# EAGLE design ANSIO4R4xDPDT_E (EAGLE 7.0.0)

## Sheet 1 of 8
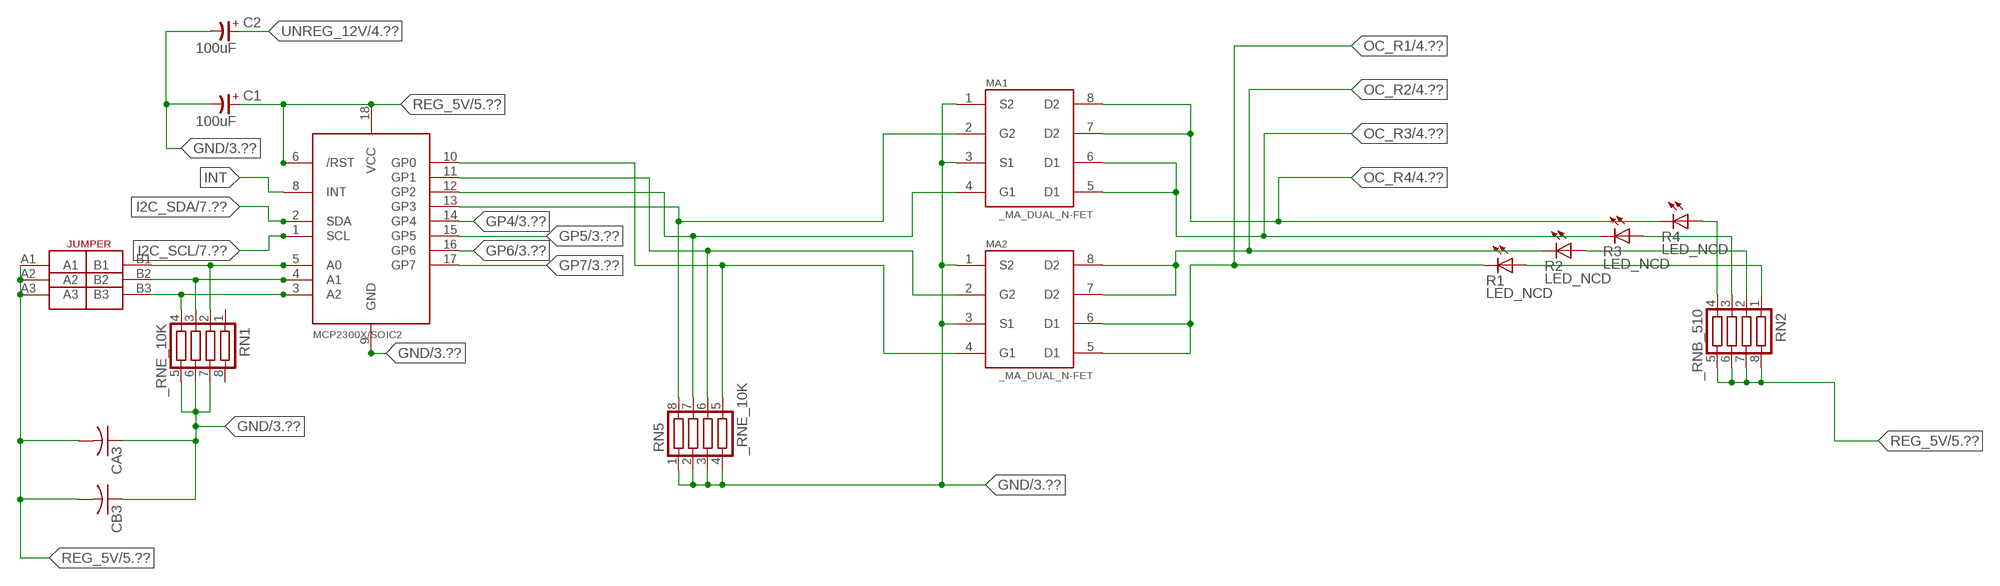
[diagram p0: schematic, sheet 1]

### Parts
C1  100uF  CP-E-025X060  [E-025X060]
C2  100uF  CP-E-025X060  [E-025X060]
CA3  CC1206KRX7R9BB104C1206K  [CC1206KRX7R9BB104]
CB3  TMK316F106ZL-TC1206K  [TMK316F106ZL-T]
IC2  MCP2300X/SO  [SO18W]
MA1  _MA_DUAL_N-FET  [_MA_DUAL_N-FET]
MA2  _MA_DUAL_N-FET  [_MA_DUAL_N-FET]
R1  LED_NCD  [CHIPLED_0603]
R2  LED_NCD  [CHIPLED_0603]
R3  LED_NCD  [CHIPLED_0603]
R4  LED_NCD  [CHIPLED_0603]
RN1  _RNE_10K  [RNE]
RN2  _RNB_510  [RNB]
RN5  _RNE_10K  [RNE]
U$18  JUMPER_3X2  [JUMPER_3X2]

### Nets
GND: C1.- C2.- CA3.1 CB3.1 IC2.9(GND) MA1.1(S2) MA1.3(S1) MA2.1(S2) MA2.3(S1) RN1.5 RN1.6 RN1.7 RN5.1 RN5.2 RN5.3 RN5.4 ; also sheet 3,5,6,7,8
GP4: IC2.14(GP4) ; also sheet 3
GP5: IC2.15(GP5) ; also sheet 3
GP6: IC2.16(GP6) ; also sheet 3
GP7: IC2.17(GP7) ; also sheet 3
I2C_SCL: IC2.1(SCL) ; also sheet 7,8
I2C_SDA: IC2.2(SDA) ; also sheet 7,8
INT: IC2.8(INT)
N$6: IC2.5(A0) RN1.2 U$18.B1
N$7: IC2.4(A1) RN1.3 U$18.B2
N$8: IC2.3(A2) RN1.4 U$18.B3
N$20: IC2.13(GP3) MA1.2(G2) RN5.8
N$21: IC2.12(GP2) MA1.4(G1) RN5.7
N$22: IC2.11(GP1) MA2.2(G2) RN5.6
N$23: IC2.10(GP0) MA2.4(G1) RN5.5
N$29: R4.A RN2.4
N$30: R3.A RN2.3
N$31: R2.A RN2.2
N$32: R1.A RN2.1
OC_R1: MA2.5(D1) MA2.6(D1) R1.C ; also sheet 4
OC_R2: MA2.7(D2) MA2.8(D2) R2.C ; also sheet 4
OC_R3: MA1.5(D1) MA1.6(D1) R3.C ; also sheet 4
OC_R4: MA1.7(D2) MA1.8(D2) R4.C ; also sheet 4
REG_5V: C1.+ CA3.2 CB3.2 IC2.6(/RST) IC2.18(VCC) RN2.5 RN2.6 RN2.7 RN2.8 U$18.A1 U$18.A2 U$18.A3 ; also sheet 5,6,7,8
UNREG_12V: C2.+ ; also sheet 4,5
Unconnected: RN1.1 RN1.8

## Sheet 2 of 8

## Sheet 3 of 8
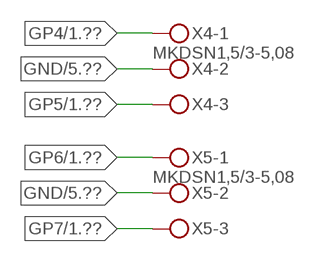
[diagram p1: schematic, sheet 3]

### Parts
X4  MKDSN1,5/3-5,08  [MKDSN1,5/3-5,08]
X5  MKDSN1,5/3-5,08  [MKDSN1,5/3-5,08]

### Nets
GND: X4.2 X5.2 ; also sheet 1,5,6,7,8
GP4: X4.1 ; also sheet 1
GP5: X4.3 ; also sheet 1
GP6: X5.1 ; also sheet 1
GP7: X5.3 ; also sheet 1

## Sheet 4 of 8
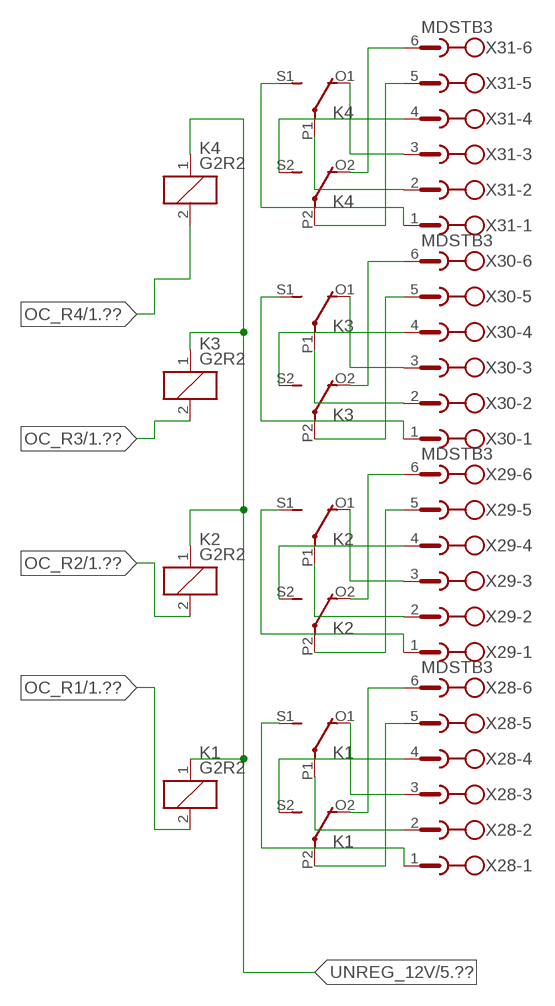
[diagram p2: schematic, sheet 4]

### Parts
K1  G2R2  [G2R2]
K2  G2R2  [G2R2]
K3  G2R2  [G2R2]
K4  G2R2  [G2R2]
X28  MDSTB3  [MDSTB3]
X29  MDSTB3  [MDSTB3]
X30  MDSTB3  [MDSTB3]
X31  MDSTB3  [MDSTB3]

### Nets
N$9: K3.P2(3:COM) X30.5
N$10: K3.O2(3:NC) X30.6
N$11: K4.P2(3:COM) X31.5
N$12: K4.O2(3:NC) X31.6
N$13: K3.S2(3:NO) X30.4
N$14: K4.S2(3:NO) X31.4
N$15: K3.O1(2:NC) X30.3
N$16: K4.O1(2:NC) X31.3
N$17: K4.P1(2:COM) X31.2
N$18: K3.P1(2:COM) X30.2
N$19: K3.S1(2:NO) X30.1
N$24: K4.S1(2:NO) X31.1
N$203: K1.P2(3:COM) X28.5
N$204: K1.O2(3:NC) X28.6
N$205: K1.S2(3:NO) X28.4
N$206: K1.P1(2:COM) X28.2
N$207: K1.O1(2:NC) X28.3
N$208: K1.S1(2:NO) X28.1
N$209: K2.P2(3:COM) X29.5
N$210: K2.O2(3:NC) X29.6
N$211: K2.S2(3:NO) X29.4
N$212: K2.S1(2:NO) X29.1
N$213: K2.P1(2:COM) X29.2
N$214: K2.O1(2:NC) X29.3
OC_R1: K1.2(1:C2) ; also sheet 1
OC_R2: K2.2(1:C2) ; also sheet 1
OC_R3: K3.2(1:C2) ; also sheet 1
OC_R4: K4.2(1:C2) ; also sheet 1
UNREG_12V: K1.1(1:C1) K2.1(1:C1) K3.1(1:C1) K4.1(1:C1) ; also sheet 1,5

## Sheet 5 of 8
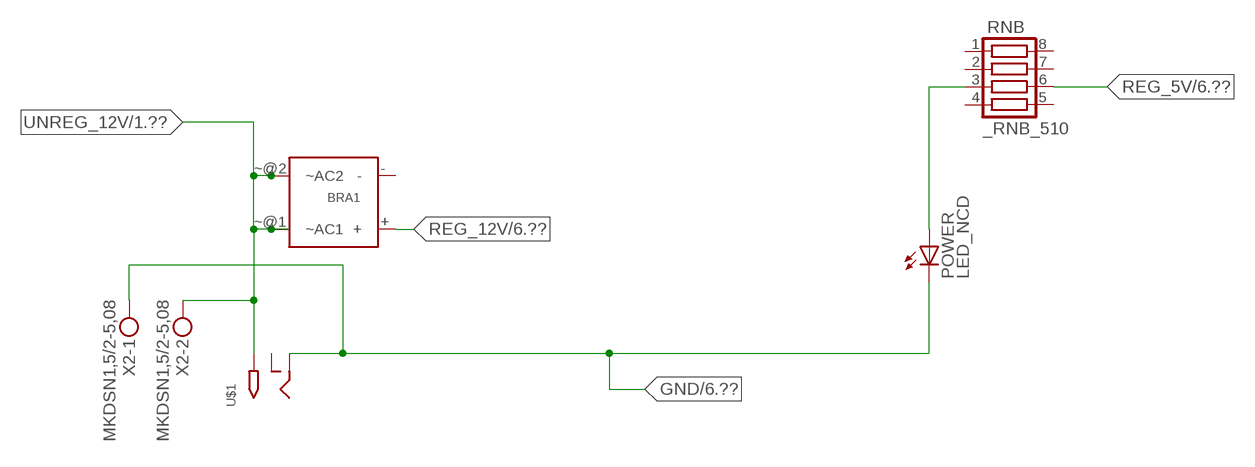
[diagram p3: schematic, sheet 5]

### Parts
BRA1  MB2S_  [MB2S]
POWER  LED_NCD  [CHIPLED_0603]
RNB  _RNB_510  [RNB]
U$1  2.1MMJACK  [PJ-102A]
X2  MKDSN1,5/2-5,08  [MKDSN1,5/2-5,08]

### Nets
GND: POWER.C U$1.RING X2.1 ; also sheet 1,3,6,7,8
N$2: POWER.A RNB.3
REG_5V: RNB.6 ; also sheet 1,6,7,8
REG_12V: BRA1.+ ; also sheet 6
UNREG_12V: BRA1.~@1(~AC1) BRA1.~@2(~AC2) U$1.TIP X2.2 ; also sheet 1,4
Unconnected: BRA1.- RNB.1 RNB.2 RNB.4 RNB.5 RNB.7 RNB.8 U$1.RING_SW

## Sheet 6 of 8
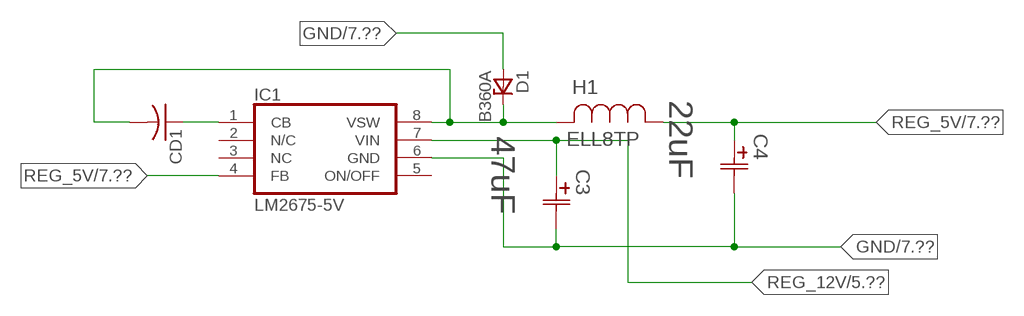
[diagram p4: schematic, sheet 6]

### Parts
C3  47uF  490-5463-6-NDCAP  [C2917(7343)-Y]
C4  22uF  490-5463-6-NDCAP  [C2917(7343)-Y]
CD1  _CD_10NF_50VC1206K  [_CD_10NF_50V]
D1  B360A  [DO214AC_ZENER]
H1  ELL8TP  [IND_ELL8TP]
IC1  LM2675-5V  LM2675  [SO-8]

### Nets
GND: C3.2(C2) C4.2(C2) D1.A IC1.6(GND) ; also sheet 1,3,5,7,8
N$1: CD1.2 D1.C H1.2 IC1.8(VSW)
N$3: CD1.1 IC1.1(CB)
REG_5V: C4.1(C1) H1.1 IC1.4(FB) ; also sheet 1,5,7,8
REG_12V: C3.1(C1) IC1.7(VIN) ; also sheet 5
Unconnected: IC1.2(N/C) IC1.5(ON/OFF)

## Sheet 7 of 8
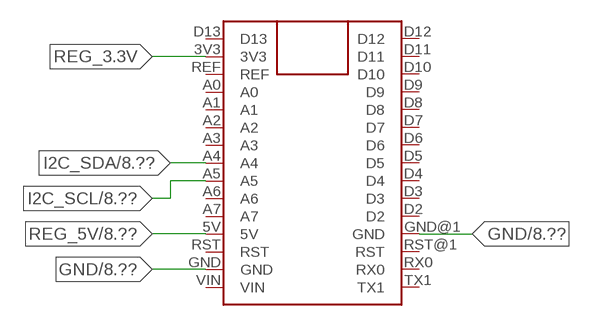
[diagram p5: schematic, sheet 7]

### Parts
FOR_NANO  ARDUINO_NANO  [ARDUINO_NANO]

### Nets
GND: FOR_NANO.GND FOR_NANO.GND@1(GND) ; also sheet 1,3,5,6,8
I2C_SCL: FOR_NANO.A5 ; also sheet 1,8
I2C_SDA: FOR_NANO.A4 ; also sheet 1,8
REG_3.3V: FOR_NANO.3V3
REG_5V: FOR_NANO.5V ; also sheet 1,5,6,8
Unconnected: FOR_NANO.A0 FOR_NANO.A1 FOR_NANO.A2 FOR_NANO.A3 FOR_NANO.A6 FOR_NANO.A7 FOR_NANO.D2 FOR_NANO.D3 FOR_NANO.D4 FOR_NANO.D5 FOR_NANO.D6 FOR_NANO.D7 FOR_NANO.D8 FOR_NANO.D9 FOR_NANO.D10 FOR_NANO.D11 FOR_NANO.D12 FOR_NANO.D13 FOR_NANO.REF FOR_NANO.RST FOR_NANO.RST@1(RST) FOR_NANO.RX0 FOR_NANO.TX1 FOR_NANO.VIN

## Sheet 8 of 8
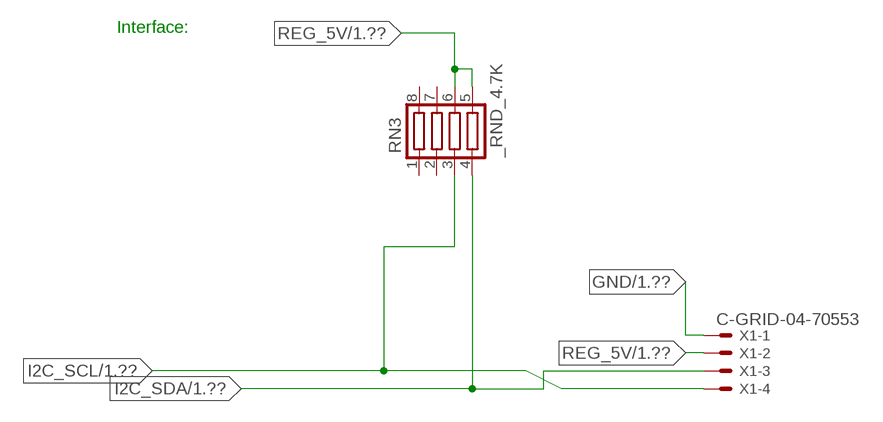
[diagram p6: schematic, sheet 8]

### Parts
RN3  _RND_4.7K  [RND]
X1  C-GRID-04-70553  [70553-04]

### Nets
GND: X1.1 ; also sheet 1,3,5,6,7
I2C_SCL: RN3.3 X1.4 ; also sheet 1,7
I2C_SDA: RN3.4 X1.3 ; also sheet 1,7
REG_5V: RN3.5 RN3.6 X1.2 ; also sheet 1,5,6,7
Unconnected: RN3.1 RN3.2 RN3.7 RN3.8

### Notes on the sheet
- Interface:

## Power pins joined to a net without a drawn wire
NC: IC1.3(NC)

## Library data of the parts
BRA1 = NCD_ULTIMATE_LIBRARY:MB2S: Bridge Rectifier BRA MB2S 200V 500ma Digikey MB2S-TPMSTR-ND/MB2S-TP
C1 C2 = NCD_ULTIMATE_LIBRARY:CP-: Capacitors All Kinds POLARIZED CAP
C3 C4 = NCD_ULTIMATE_bhaskar:490-5463-6-ND: NCD CAP
CA3 = NCD_ULTIMATE_LIBRARY:CC1206KRX7R9BB104: Capacitor CA .1uF 50V SMT C1206K CC1206KRX7R9BB104
CB3 = NCD_ULTIMATE_LIBRARY:TMK316F106ZL-T: Capacitor CB 10uF SMT 1206 TMK316F106ZL-T
CD1 = NCD_ULTIMATE_LIBRARY:_CD_10NF_50V: Capacitor 10nF SMT
D1 = NCD_ULTIMATE_bhaskar:B360A: NCD DIODE B350A/B360A
FOR_NANO = NCD_ULTIMATE_CONNECTORS:ARDUINO_NANO
H1 = NCD_ULTIMATE_bhaskar:ELL8TP: NCD coil
IC1 = NCD_ULTIMATE_bhaskar:LM2675: LM2675 NCD http://www.ti.com/lit/ds/symlink/lm2675.pdf
IC2 = NCD_ULTIMATE_LIBRARY:MCP2300X: Semiconductor Port Expander I/O 8-Bit I2C MCP23008 Inexpensive i2c i/o expander - 8 general purpose i/o pins with optional pullups
K1-K4 = NCD_ULTIMATE_LIBRARY:G2R2: RELAY 2 x switch, Omron
MA1 MA2 = NCD_ULTIMATE_LIBRARY:_MA_DUAL_N-FET: FET Dual N-Channel 8-SOIC NMOSFET Digikey 785-1064-2-ND/AO4842
POWER = NCD_ULTIMATE_bhaskar:LED_NCD
R1-R4 = NCD_ULTIMATE_LIBRARY:LED_NCD: LED Digikey 754-1132-2-ND/APT2012SRCPRV
RN1 RN5 = NCD_ULTIMATE_LIBRARY:_RNE_10K: Resistor Array RNE SMT 10K x 4 Single Resistor Source: http://www.ctscorp.com/components/Datasheets/CTSChipArrayDs.pdf Digikey 742C083103JPTR-ND/742C083103JP; OC_FARNELL: unknown; OC_NEWARK: unknown
RN2 RNB = NCD_ULTIMATE_LIBRARY:_RNB_510: Resistor Array RNB SMT 510 x 4 Single Resistor Source: http://www.ctscorp.com/components/Datasheets/CTSChipArrayDs.pdf Digikey 742C083511JPTR-ND/ 742C083511JP; OC_FARNELL: unknown; OC_NEWARK: unknown
RN3 = NCD_ULTIMATE_LIBRARY:_RND_4.7K: Resistor Array RND SMT 4.7K x 4 Single Resistor Source: http://www.ctscorp.com/components/Datasheets/CTSChipArrayDs.pdf Digikey 742C083472JPTR-ND/742C083472JP; OC_FARNELL: unknown; OC_NEWARK: unknown
U$1 = NCD_ULTIMATE_CONNECTORS:2.1MMJACK: 2.1mm x 5.5mm DC jack with internal switch. Digikey part #PJ-102A, 4UCON part #05537 By microbuilder.eu
U$18 = NCD_ULTIMATE_CONNECTORS:JUMPER_3X2
X1 = NCD_ULTIMATE_CONNECTORS:C-GRID-04: CONNECTOR 4-Pos I2C wire to board 2.54 mm (0.100") pitch header Digikey WM1342-ND/0015912045; OC_FARNELL: unknown; OC_NEWARK: unknown
X2 = NCD_ULTIMATE_CONNECTORS:MKDSN1,5/2-5,08: MKDSN 1,5/ 2-5,08 Printklemme
X4 X5 = NCD_ULTIMATE_CONNECTORS:MKDSN1,5/3-5,08: MKDSN 1,5/ 3-5,08 Printklemme Nennstrom: 13,5 A Nennspannung: 250 V Rastermaß: 5,08 mm Polzahl: 3 Anschlussart: Schraubanschluss Montage: Löten Anschlussrichtung Leiter/Platine: 0 ° Artikelnummer: 1729131 Source: http://eshop.phoenixcontact.com .. 1729131.pdf
X28-X31 = NCD_ULTIMATE_LIBRARY:MDSTB3: PHOENIX

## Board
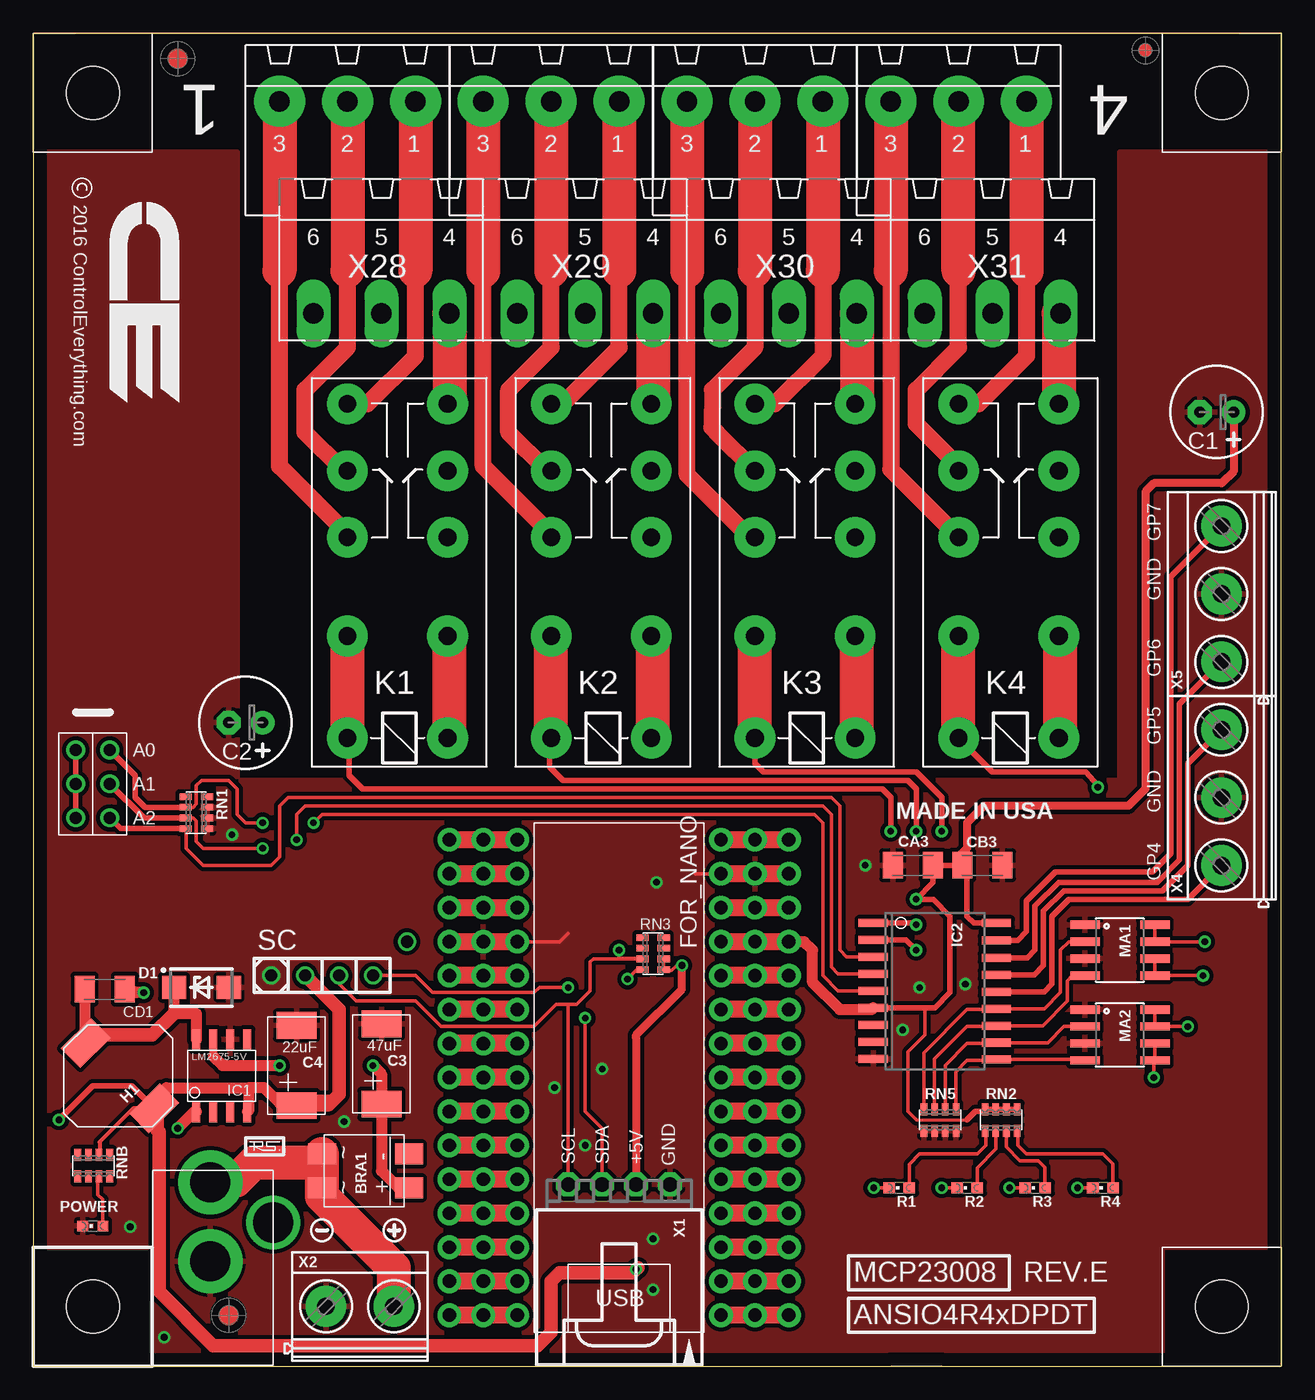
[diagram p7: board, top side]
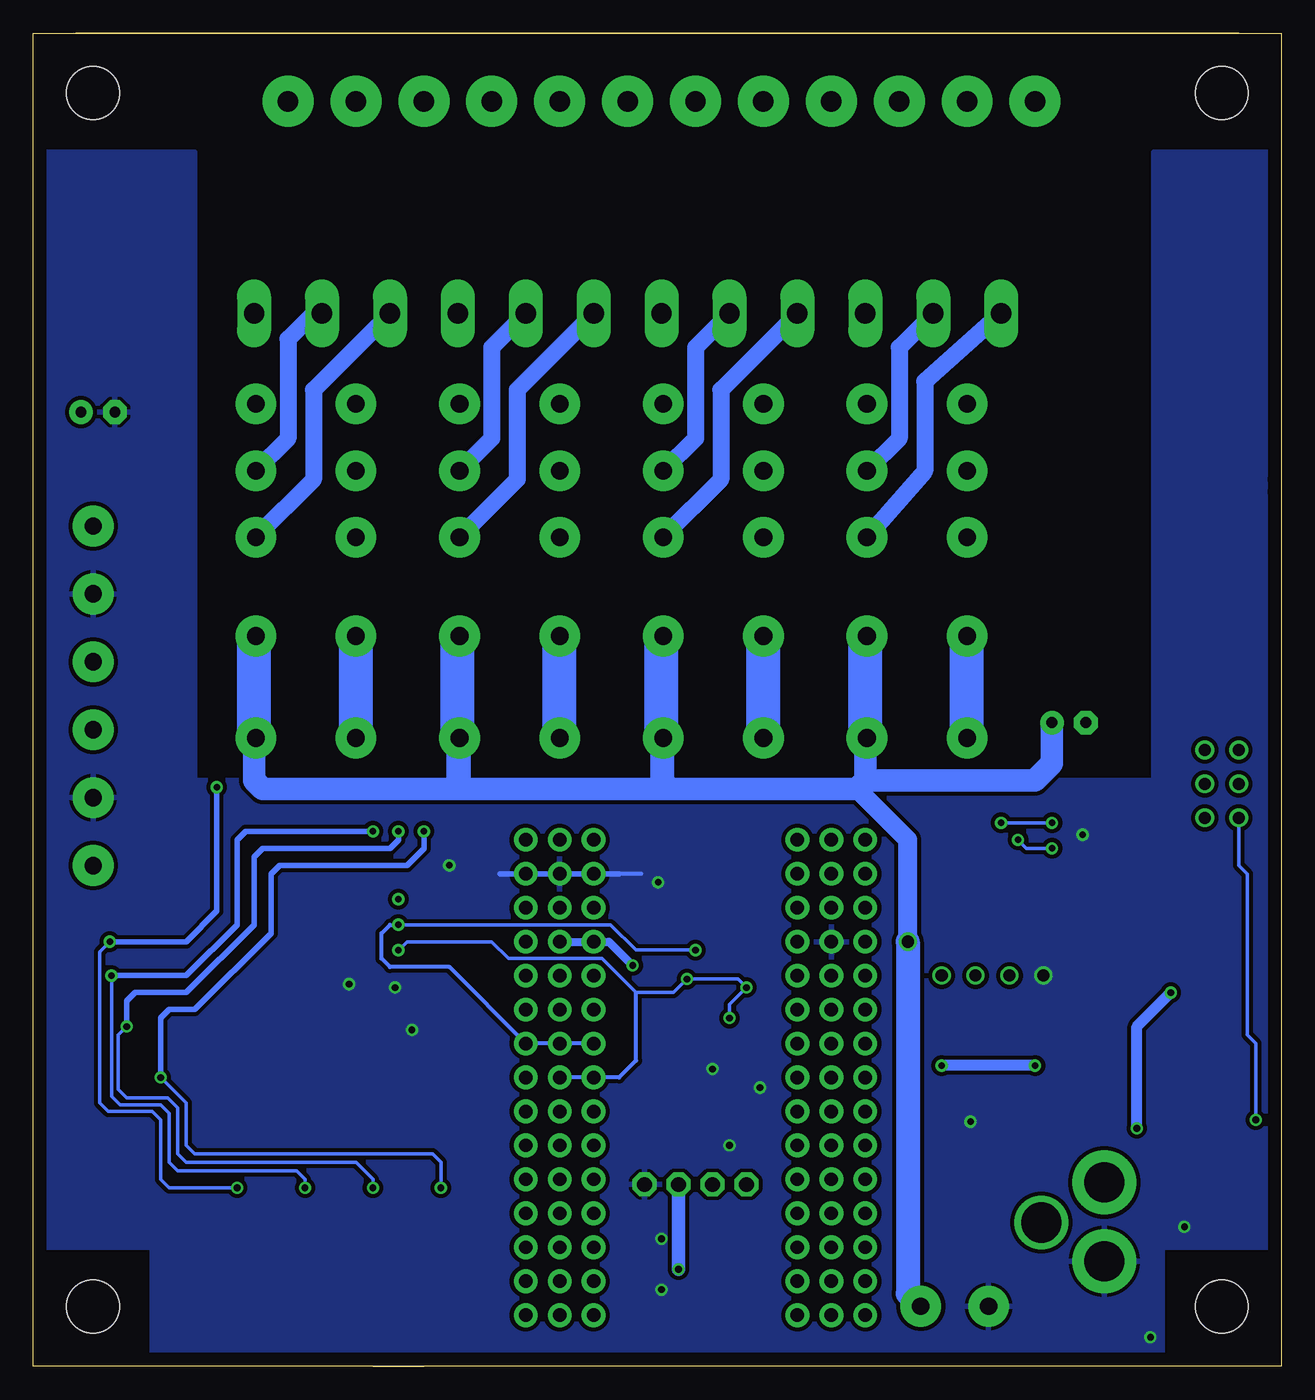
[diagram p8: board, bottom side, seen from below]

Size 93.34 x 99.7 mm. Coordinates in mm from the lower left corner, seen from the top.
Outline: 0,66.34 0,65.41
Outline: 0,65.41 0,0 64.14,0
Outline: 64.14,0 93.34,0 93.34,99.7 0,99.7 0,65.41
Outline: 3.17,99.7 90.17,99.7
Outline: 67.94,0 64.14,0
Copper layers (1*16): Top 0.035mm / dielectric 1.5mm / Bottom 0.035mm
Design rules "default": minimum track width 10mil, minimum drill 24mil, track to track 8mil, track to pad 8mil, pad to pad 8mil, via to via 8mil, smd to smd 8mil, copper to edge 40mil, drill to drill 8mil, minimum pad ring 10mil, minimum via ring 8mil, stop-mask expansion 4mil, vias tented up to drill 0mil, thermal gap 10mil
Holes 3.96 mm at 4.45,4.45 4.45,4.45 4.45,4.45

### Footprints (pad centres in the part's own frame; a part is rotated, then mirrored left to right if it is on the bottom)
MB2S = smd 1.55 x 2.1: + 0,-6.5; - 2.54,-6.5; ~@1 0,0; ~@2 2.54,0
E-025X060 = drill 0.813 pad 1.778: + -1.27,0 | drill 0.813 pad 1.778 octagon: - 1.27,0
C2917(7343)-Y = smd 2 x 3: 1 -3,0; 2 3,0
CC1206KRX7R9BB104 = smd 1.5 x 2: 1 -1.5,0; 2 1.5,0
TMK316F106ZL-T = smd 1.5 x 2: 1 -1.5,0; 2 1.5,0
_CD_10NF_50V = smd 1.5 x 2: 1 -1.5,0; 2 1.5,0
DO214AC_ZENER = smd 1.8 x 1.7: A 2.05,0; C -2.05,0
ARDUINO_NANO = drill 1 pad 1.778: 3V1 -2.54,-2.54; 3V3 0,-2.54; 5V 0,-27.94; 5V1 -2.54,-27.94; A0 0,-7.62; A1 0,-10.16; A2 0,-12.7; A3 0,-15.24; A4 0,-17.78; A5 0,-20.32; A6 0,-22.86; A7 0,-25.4; A8 -2.54,-7.62; A9 -2.54,-10.16; A10 -2.54,-12.7; A11 -2.54,-15.24; A12 -2.54,-17.78; A13 -2.54,-20.32; A14 -2.54,-22.86; A15 -2.54,-25.4; D1 -2.54,0; D2 20.32,-25.4; D3 20.32,-22.86; D4 20.32,-20.32; D5 20.32,-17.78; D6 20.32,-15.24; D7 20.32,-12.7; D8 20.32,-10.16; D9 20.32,-7.62; D10 20.32,-5.08; D11 20.32,-2.54; D12 20.32,0; D13 0,0; D14 22.86,0; D15 22.86,-2.54; D16 22.86,-5.08; D17 22.86,-7.62; D18 22.86,-10.16; D19 22.86,-12.7; D20 22.86,-15.24; D21 22.86,-17.78; D22 22.86,-20.32; D23 22.86,-22.86; D24 22.86,-25.4; GND 0,-33.02; GND1 -2.54,-33.02; GND@1 20.32,-27.94; GND@2 22.86,-27.94; P$16 2.54,0; P$17 2.54,-2.54; P$18 2.54,-5.08; P$19 2.54,-7.62; P$20 2.54,-10.16; P$21 2.54,-12.7; P$22 2.54,-15.24; P$23 2.54,-17.78; P$24 2.54,-20.32; P$25 2.54,-22.86; P$26 2.54,-25.4; P$27 2.54,-27.94; P$28 2.54,-30.48; P$29 2.54,-33.02; P$30 2.54,-35.56; P$31 17.78,0; P$32 17.78,-2.54; P$33 17.78,-5.08; P$34 17.78,-7.62; P$35 17.78,-10.16; P$36 17.78,-12.7; P$37 17.78,-15.24; P$38 17.78,-17.78; P$39 17.78,-20.32; P$40 17.78,-22.86; P$41 17.78,-25.4; P$42 17.78,-27.94; P$43 17.78,-30.48; P$44 17.78,-33.02; P$45 17.78,-35.56; REF 0,-5.08; REF1 -2.54,-5.08; RST 0,-30.48; RST1 -2.54,-30.48; RST@1 20.32,-30.48; RST@2 22.86,-30.48; RX0 20.32,-33.02; RX1 22.86,-33.02; TX1 20.32,-35.56; TX2 22.86,-35.56; VIN 0,-35.56; VIN1 -2.54,-35.56
IND_ELL8TP = smd 2.054 x 3.2 rotated 45: 1 -2.442,-2.696; 2 2.442,2.442
SO-8 = smd 0.6 x 1.55: 1 -1.905,-2.69; 2 -0.635,-2.69; 3 0.635,-2.69; 4 1.905,-2.69; 5 1.905,2.71; 6 0.635,2.71; 7 -0.635,2.71; 8 -1.905,2.71
SO18W = smd 0.6 x 2.2: 1 -4.445,-4.6; 2 -3.175,-4.6; 3 -1.905,-4.6; 4 -0.635,-4.6; 5 0.635,-4.6; 6 1.905,-4.6; 7 3.175,-4.6; 8 4.445,-4.6; 9 5.715,-4.6; 10 5.775,4.6; 11 4.505,4.6; 12 3.235,4.6; 13 1.965,4.6; 14 0.695,4.6; 15 -0.575,4.6; 16 -1.845,4.6; 17 -3.145,4.6; 18 -4.445,4.6
G2R2 = drill 1.321 pad 3.048: 1 -2.54,-3.683; 2 -2.54,3.81; 3 5.08,-3.683; 4 5.08,3.81; O1 12.471,3.81; O2 12.471,-3.683; P1 17.45,3.81; P2 17.45,-3.683; S1 22.454,3.81; S2 22.454,-3.683
_MA_DUAL_N-FET = smd 0.61 x 2.21: 1 -1.905,-2.616; 2 -0.635,-2.616; 3 0.635,-2.616; 4 1.905,-2.616; 5 1.905,2.616; 6 0.635,2.616; 7 -0.635,2.616; 8 -1.905,2.616
CHIPLED_0603 = smd 0.8 x 0.8: A 0,-0.75; C 0,0.75
CHIPLED_0603' = smd 0.8 x 0.876: A 0,-0.75; C 0,0.75
RNE = smd 0.5 x 0.9: 1 -1.2,-0.8; 2 -0.4,-0.8; 3 0.4,-0.8; 4 1.2,-0.8; 5 1.2,0.8; 6 0.4,0.8; 7 -0.4,0.8; 8 -1.2,0.8
RNB = smd 0.5 x 0.9: 1 -1.2,-0.8; 2 -0.4,-0.8; 3 0.4,-0.8; 4 1.2,-0.8; 5 1.2,0.8; 6 0.4,0.8; 7 -0.4,0.8; 8 -1.2,0.8
RND = smd 0.5 x 0.9: 1 -1.2,-0.8; 2 -0.4,-0.8; 3 0.4,-0.8; 4 1.2,-0.8; 5 1.2,0.8; 6 0.4,0.8; 7 -0.4,0.8; 8 -1.2,0.8
PJ-102A = drill 3 pad 4.8: RING 0.1,-3.39; TIP 0.1,-9.29 | drill 3 pad 3.251: RING_SW -4.6,-6.29
PCB_MOUNTING_HOLE = hole 3.962: 4.445,4.445
JUMPER_3X2 = drill 0.9: A1 0,5.08; A2 0,2.54; A3 0,0; B1 2.54,5.08; B2 2.54,2.54; B3 2.54,0
70553-04 = drill 1.1 pad 1.778 octagon: 1 -3.81,-7.62; 2 -1.27,-7.62; 3 1.27,-7.62; 4 3.81,-7.62
MKDSN1,5/2-5,08 = drill 1.3 pad 3.048: 1 -2.561,0.025; 2 2.519,0.025
MKDSN1,5/3-5,08 = drill 1.3 pad 3.048: 1 -7.641,0.025; 2 -2.561,0.025; 3 2.519,0.025
MDSTB3 = drill 1.524 pad 3.81: 1 -3.81,-10.795; 2 1.27,-10.795; 3 6.35,-10.795 | drill 1.524 pad 2.54 long: 4 -6.35,5.08; 5 -1.27,5.08; 6 3.81,5.08

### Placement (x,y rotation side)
BRA1  21.59,13.34 90 top
C1  88.52,71.37 180 top
C2  15.88,48.13 180 top
C3  26.04,22.61 90 top
C4  19.68,22.48 90 top
CA3  65.79,37.47 0 top
CB3  70.99,37.47 180 top
CD1  5.33,28.19 180 top
D1  12.57,28.32 0 top
FOR_NANO  53.98,3.81 180 top
H1  6.35,21.72 90 top
IC1  14.1,21.72 0 top
IC2  67.44,28.7 270 top
K1  27.3,49.53 90 top
K2  42.55,49.53 90 top
K3  57.78,49.53 90 top
K4  73.03,49.53 90 top
MA1  81.28,31.12 270 top
MA2  81.28,24.77 270 top
POWER  4.45,10.48 90 top
R1  LED_NCD  [CHIPLED_0603']  64.77,13.34 90 top
R2  LED_NCD  [CHIPLED_0603']  69.85,13.34 90 top
R3  LED_NCD  [CHIPLED_0603']  74.93,13.34 90 top
R4  LED_NCD  [CHIPLED_0603']  80.01,13.34 90 top
RN1  12.19,41.4 270 top
RN2  72.39,18.41 0 top
RN3  46.35,30.86 270 top
RN5  67.82,18.41 0 top
RNB  4.51,14.99 0 top
U$1  13.34,4.45 180 top
U$2  [VISION_REF15]  14.61,3.81 0 top
U$3  [ICON_MINUS]  21.59,10.16 180 top
U$4  PCB_MOUNTING_HOLE  [PCB_MOUNTING_HOLE]  93.34,90.81 90 top
U$5  [ICON_PLUS]  26.99,10.16 90 top
U$6  PCB_MOUNTING_HOLE  [PCB_MOUNTING_HOLE]  93.34,0 90 top
U$11  PCB_MOUNTING_HOLE  [PCB_MOUNTING_HOLE]  8.89,90.81 90 top
U$15  [VISION_REF15]  10.79,97.79 270 top
U$18  3.17,41.02 0 top
U$19  [VISION_REF10]  83.19,98.43 0 top
U$21  [ICON_USA]  64.52,40.89 0 top
X1  43.81,5.97 180 top
X2  24.45,4.45 0 top
X4  88.9,45.09 90 top
X5  88.9,60.32 90 top
X28  24.77,83.82 180 top
X29  40.01,83.82 180 top
X30  55.24,83.82 180 top
X31  70.48,83.82 180 top

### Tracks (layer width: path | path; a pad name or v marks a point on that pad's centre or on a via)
GND  (via drill 0.5, 0.9)
  Top 0.254: 36.2,31.75 39.37,31.75 40.01,32.38 | FOR_NANO.GND@1 32.38,31.75 | 49.53,36.83 56.52,36.83 56.77,36.83
  Top 1.016: X1.1 47.62,13.49
  Bottom 0.254: 51.44,36.83 FOR_NANO.GND
  Bottom 0.305: 47.88,36.83 49.53,36.83 51.44,36.83
  Bottom 0.406: 49.53,36.83 58.42,36.83
  other vias: 14.86,39.75 65.02,25.15 62.23,37.47 9.78,2.16 17.78,29.21 41.27,16.51 46.35,9.53 46.61,36.2 46.35,5.71 42.55,22.23 38.99,20.83 7.24,10.41 66.29,28.32 69.72,28.58 23.24,18.29
  pour Bottom (isolate 0.305): -3.81,8.89 8.89,8.89 8.89,0 84.45,0 84.45,8.89 92.71,8.89 92.71,90.81 81.28,90.81 81.28,43.81 9.53,43.81 9.53,90.81 -3.81,90.81
  pour Top (isolate 0.305): -8.26,8.89 8.89,8.89 8.89,0 84.45,0 84.45,8.89 92.71,8.89 92.71,90.81 81.28,90.81 81.28,43.81 15.24,43.81 15.24,90.81 -8.26,90.81
GP4
  Top 0.406: IC2.14 75.63,28.01 76.2,28.58 76.2,33.66 77.47,34.92 86.36,34.92 X4.1
GP5
  Top 0.406: IC2.15 74.87,29.28 75.56,29.97 75.56,34.04 77.09,35.56 84.45,35.56 86.36,37.47 86.36,45.09 X4.3
GP6
  Top 0.406: IC2.16 74.36,30.55 74.93,31.12 74.93,34.42 76.71,36.2 84.07,36.2 85.72,37.85 85.72,49.53 X5.1
GP7
  Top 0.406: IC2.17 73.63,31.85 74.3,32.51 74.3,34.8 76.45,36.96 83.69,36.96 85.09,38.35 85.09,59.06 X5.3
I2C_SCL  (via drill 0.5, 0.9)
  Top 0.254: 40.01,27.05 40.64,27.05 41.64,28.05 41.64,29.48 41.66,29.5 41.66,30.23 41.89,30.46 RN3.3 45.54,30.48 43.81,30.48 v43.81,31.12 | 40.01,27.05 39.12,27.05 37.47,25.4 30.48,25.4 28.57,27.3 24.13,27.3 22.86,28.58 v22.86,29.21 | X1.4 40.01,27.05
  Top 0.406: IC2.1 65.91,33.15 v66.04,33.02
  Bottom 0.254: v43.81,31.12 48.26,31.12 50.16,33.02 v66.04,33.02
  Bottom 0.305: v66.04,33.02 66.67,33.02 67.31,32.38 67.31,30.48 66.67,29.84 62.23,29.84 56.52,24.13 FOR_NANO.A5 51.44,24.13
I2C_SDA  (via drill 0.5, 0.9)
  Top 0.254: RN3.4 45.16,29.66 v44.45,28.96 | 40,28.33 v40.01,28.32 37.85,28.32 37.47,27.94 29.84,27.94 28.57,29.21 v25.4,29.21 | X1.3 42.55,17.78 41.27,19.05 v41.27,26.04
  Top 0.406: IC2.2 65.28,31.88 v66.04,31.12
  Bottom 0.254: v66.04,31.12 65.41,31.75 59.05,31.75 57.78,30.48 50.8,30.48 48.26,27.94 45.47,27.94 v44.45,28.96 40.64,28.96 v40.01,28.32 41.27,27.05 v41.27,26.04
  Bottom 0.305: 48.26,27.94 48.26,22.86 49.53,21.59 FOR_NANO.A4
N$1
  Top 0.813: H1.2 3.88,24.77 | D1.C 10.52,26.4 12.19,26.38 IC1.8 | CD1.2 3.83,24.15 4.45,24.77
  Top 1.016: 3.88,24.77 4.45,24.77 8.89,24.77 10.52,26.4
N$2
  Top 0.254: POWER.A 5.2,12.46 4.83,12.83 4.83,14.1 RNB.3
  Top 0.406: 4.95,14.14 RNB.3
N$3  (via drill 0.5)
  Top 0.813: IC1.1 12.04,19.03 v10.79,17.78 | v8.26,27.94 7.72,27.94 CD1.1
  Bottom 0.813: v10.79,17.78 10.79,25.4 v8.26,27.94
N$6  (via drill 0.5)
  Top 0.254: IC2.5 60.2,28.07 59.05,29.21 59.05,40.64 58.42,41.27 21.59,41.27 v20.95,40.64 | v17.14,40.64 15.88,40.64 15.24,41.27 15.24,43.18 14.61,43.81 12.57,43.81 12.19,43.43 12.19,42.04 11.94,41.78 11.41,41.78 RN1.2
  Top 0.406: RN1.2 8.36,41.8 7.62,42.55 7.62,44.2 U$18.B1
  Bottom 0.254: v20.95,40.64 v17.14,40.64
N$7  (via drill 0.5)
  Top 0.254: IC2.4 60.2,29.34 59.69,29.84 59.69,41.27 59.05,41.91 20.32,41.91 19.68,41.27 v19.68,39.37 | v17.14,38.73 12.7,38.73 12.19,39.24 12.19,40.77 11.94,41.02 11.41,41.02 RN1.3
  Top 0.406: RN1.3 8.27,41 U$18.B2
  Bottom 0.254: v19.68,39.37 19.05,38.73 v17.14,38.73
N$8
  Top 0.254: IC2.3 60.83,30.61 60.33,31.12 60.33,41.91 59.69,42.55 19.05,42.55 18.41,41.91 18.41,38.1 17.78,37.47 12.7,37.47 11.43,38.73 11.43,40.16 RN1.4
  Top 0.406: RN1.4 6.53,40.2 U$18.B3
N$9
  Bottom 1.27: X30.5 59.05,76.2 59.05,69.39 K3.P2
N$10
  Bottom 1.27: X30.6 57.15,73.03 57.15,66.32 K3.O2
N$11
  Bottom 1.27: X31.5 72.39,78.74 74.3,76.84 74.3,69.39 K4.P2
N$12
  Bottom 1.27: X31.6 72.39,73.03 72.39,66.32 K4.O2
N$13
  Top 2.54: X30.4 61.59,72.11 K3.S2
N$14
  Top 2.54: X31.4 76.71,78.74 K4.S2
N$15
  Top 1.27: K3.O1 53.57,62 48.9,66.67 48.9,81.92
  Top 2.54: X30.3 48.9,81.92
N$16
  Top 1.27: 64.14,81.92 64.14,67.08 K4.O1
  Top 2.54: X31.3 64.14,81.92
N$17
  Top 1.27: K4.P1 69.22,67.31 66.04,70.48 66.04,73.03 69.22,76.2 69.22,81.92
  Top 2.54: 69.22,81.92 X31.2
N$18
  Top 1.27: 53.98,81.92 53.98,76.2 50.8,73.03 50.75,70.23 51.1,69.85 K3.P1
  Top 2.54: X30.2 53.98,81.92
N$19
  Top 1.27: 59.05,81.92 59.05,75.57 55.47,71.98 K3.S1
  Top 2.54: X30.1 59.05,81.92
N$20
  Top 0.254: MA1.2 77.47,31.75 76.83,31.12 76.83,27.94 75.63,26.74 IC2.13 71.97,26.67 69.85,26.67 66.62,23.44 RN5.8
N$21
  Top 0.254: MA1.4 77.72,29.21 77.34,28.83 77.34,27.3 75.5,25.47 IC2.12 71.97,25.4 69.85,25.4 67.42,22.97 RN5.7
N$22
  Top 0.254: MA2.2 77.09,25.4 75.89,24.2 IC2.11 71.97,24.13 69.85,24.13 68.22,22.5 RN5.6
N$23
  Top 0.254: MA2.4 78.6,22.93 IC2.10 71.97,22.86 69.85,22.86 69.02,22.03 RN5.5
N$24
  Top 1.27: 74.3,81.92 74.3,75.57 70.71,71.98 K4.S1
  Top 2.54: X31.1 74.3,81.92
N$29
  Top 0.254: R4.A 80.76,15.12 80.01,15.88 74.3,15.88 73.66,16.51 73.66,17.55 RN2.4
N$30
  Top 0.254: R3.A 75.68,14.87 75.18,15.37 73.79,15.37 72.77,16.38 72.77,17.6 RN2.3
N$31
  Top 0.254: R2.A 70.6,14.85 72.01,16.26 72.01,17.6 RN2.2
N$32
  Top 0.254: R1.A 65.52,15.1 66.29,15.88 70.61,15.88 71.25,16.51 71.25,17.56 RN2.1
N$203
  Bottom 1.27: X28.5 28.57,76.2 28.57,69.39 K1.P2
N$204
  Bottom 1.27: X28.6 26.67,73.66 26.67,66.95 K1.O2
N$205
  Top 2.54: X28.4 31.11,72.11 K1.S2
N$206
  Top 1.27: K1.P1 23.19,66.98 20.32,69.85 20.32,73.03 23.5,76.2 23.5,81.92
  Top 2.54: X28.2 23.5,81.92
N$207
  Top 1.27: K1.O1 23.5,62.23 18.41,67.31 18.41,81.92
  Top 2.54: X28.3 18.41,81.92
N$208
  Top 1.27: 28.57,81.92 28.57,75.57 24.99,71.98 K1.S1
  Top 2.54: X28.1 28.57,81.92
N$209
  Bottom 1.27: X29.5 43.81,76.2 43.81,69.39 K2.P2
N$210
  Bottom 1.27: X29.6 41.91,73.03 41.91,66.32 K2.O2
N$211
  Top 2.54: X29.4 46.35,72.11 K2.S2
N$212
  Top 1.27: K2.S1 39.62,72.01 43.81,76.2 43.81,81.92
  Top 2.54: X29.1 43.81,81.92
N$213
  Top 1.27: K2.P1 38.43,66.98 35.56,69.85 35.56,73.03 38.73,76.2 38.73,81.92
  Top 2.54: X29.2 38.73,81.92
N$214
  Top 1.27: K2.O1 38.73,62.23 33.66,67.31 33.66,81.92
  Top 2.54: X29.3 33.66,81.92
OC_R1  (via drill 0.5)
  Top 0.254: R1.C v62.87,13.34 | v83.82,21.59 83.82,22.78 MA2.5 MA2.6
  Top 0.406: v64.14,40.01 64.14,42.55 63.5,43.18 24.64,43.18 23.62,44.2 23.62,46.74 23.5,46.74 K1.2
  Bottom 0.254: v62.87,13.34 62.87,15.24 63.5,15.88 81.28,15.88 81.92,16.51 81.92,19.69 v83.82,21.59
  Bottom 0.406: v83.82,21.59 83.82,26.04 83.19,26.67 81.28,26.67 75.56,32.38 75.56,36.83 74.93,37.47 65.41,37.47 64.14,38.73 v64.14,40.01
OC_R2  (via drill 0.5)
  Top 0.254: R2.C v67.94,13.34 | v86.36,25.4 MA2.7 MA2.8
  Top 0.406: v66.04,40.01 66.04,43.18 65.41,43.81 39.62,43.81 38.61,44.83 38.61,46.99 K2.2
  Bottom 0.254: v67.94,13.34 67.94,13.97 69.22,15.24 81.92,15.24 82.55,15.88 82.55,19.3 83.31,20.07 86.36,20.07 87,20.7 87,24.77 v86.36,25.4
  Bottom 0.406: v86.36,25.4 86.36,27.3 85.72,27.94 81.92,27.94 76.83,33.02 76.83,38.1 76.2,38.73 66.67,38.73 66.04,39.37 v66.04,40.01
OC_R3  (via drill 0.5)
  Top 0.254: R3.C v73.03,13.34 | v87.5,29.21 MA1.5 MA1.6
  Top 0.406: v67.94,40.01 67.94,42.55 66.04,44.45 54.61,44.45 53.98,45.09 K3.2
  Bottom 0.254: v73.03,13.34 73.03,13.97 73.66,14.61 82.55,14.61 83.19,15.24 83.19,18.92 83.82,19.56 86.87,19.56 87.5,20.19 v87.5,29.21
  Bottom 0.406: v87.5,29.21 81.92,29.21 78.11,33.02 78.11,39.37 77.47,40.01 v67.94,40.01
OC_R4  (via drill 0.5)
  Top 0.254: R4.C v78.11,13.34 | v87.63,31.75 MA1.7 MA1.8
  Top 0.406: v79.63,43.31 79.63,43.43 78.74,44.45 71.75,44.45 K4.2
  Bottom 0.254: v78.11,13.34 83.19,13.34 83.82,13.97 83.82,18.41 84.45,19.05 87.76,19.05 88.39,19.69 88.39,30.99 v87.63,31.75
  Bottom 0.406: v79.63,43.31 79.63,34.04 81.92,31.75 v87.63,31.75
REG_5V  (via drill 0.5, 0.9)
  Top 0.229: 66.04,18.41 69.85,18.41
  Top 0.254: RN3.6 RN3.5 47.23,29.59 47.75,29.59 48.13,29.97 v48.51,29.97 | 44.98,24.41 45.09,24.51 | 66.04,18.41 65.41,19.05 65.41,23.5 66.67,24.77 66.67,26.8
  Top 0.305: 62.71,26.67 60.96,26.67 | H1.1 7.46,19.27 4.95,16.76 4.95,15.83 RNB.6
  Top 0.406: U$18.A3 U$18.A2 U$18.A1 | IC2.18 70.36,33.15 69.85,33.66 69.85,37.11 CB3.2 CA3.2 67.29,36.17 v66.04,34.92 67.31,34.92 68.58,33.66 68.58,27.94 67.44,26.8 66.67,26.8 IC2.6 | 69.85,18.41 70.48,19.05 71.03,19.05 RN2.8 RN2.7 RN2.6 RN2.5 | v1.91,18.41 4.45,20.95 7.37,20.95 H1.1
  Top 0.61: C1.+ 89.79,66.93 88.9,66.04 83.82,66.04 83.19,65.41 83.19,43.18 81.92,41.91 71.12,41.91 69.85,40.64 69.85,38.73 69.22,38.1 69.22,37.74 CB3.2 | v48.51,29.97 48.51,28.19 45.09,24.77 45.09,24.51 X1.2
  Top 0.813: IC2.6 62.71,26.67 60.33,26.67 58.29,28.7 58.29,31.12 57.66,31.75 FOR_NANO.5V | 16.13,20.83 9.96,20.83 H1.1 | 16.13,20.83 17.27,20.83 18.41,19.69 20.75,19.69 C4.1 | IC1.4 16.13,19.15 16.13,20.83
  Top 1.016: H1.1 9.27,18.41 9.27,17.65 9.4,17.53 9.4,5.59 13.46,1.52 37.72,1.52 38.73,2.54 38.73,6.35 39.37,6.99 44.83,6.99 v45.09,7.24 45.21,7.37 | 22.05,19.69 22.23,19.69 22.86,20.32 22.86,26.67 v20.32,29.21
  Top 1.27: 20.75,19.69 22.05,19.69
  Bottom 0.254: U$18.A3 3.17,37.47 2.54,36.83 2.54,24.77 1.91,24.13 v1.91,18.41
  Bottom 0.61: FOR_NANO.5V 50.29,31.75 v48.51,29.97
  Bottom 1.016: v45.09,7.24 X1.2
REG_12V  (via drill 0.5)
  Top 0.61: IC1.7 13.46,23.16 | 14.1,22.48 14.15,22.48
  Top 0.813: v18.41,22.48 14.15,22.48 13.46,23.16 | v25.4,22.48 26.04,21.84 C3.1 26.04,14.61 27.3,13.34 BRA1.+
  Bottom 0.813: v18.41,22.48 v25.4,22.48
UNREG_12V  (via drill 0.9)
  Top 2.54: X2.2 26.97,7.32 21.59,12.7 BRA1.~@1 21.59,15.24 | 21.59,15.24 BRA1.~@2 | U$1.TIP 15.14,13.87 16.51,15.24 21.59,15.24
  Bottom 1.422: v27.94,31.75 27.94,39.37 31.75,43.18 | 31.11,43.81 30.48,43.81
  Bottom 1.676: 45.72,43.18 31.75,43.18 31.11,43.81 31.11,46.86 K1.1 | 45.72,43.18 46.35,43.81 46.35,46.86 K2.1 46.23,43.31 46.35,43.18 | 46.35,43.18 45.72,43.18 | 46.35,43.18 60.96,43.18 | 61.47,43.69 61.59,43.81 61.59,46.86 K3.1 61.47,43.69 | 61.47,43.69 60.96,43.18 | 60.96,43.18 76.2,43.18 76.83,43.81 76.83,46.86 K4.1 | C2.+ 17.14,45.09 18.41,43.81 30.48,43.81
  Bottom 1.778: v27.94,31.75 27.94,5.44 X2.2

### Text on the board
tNames: 1 | 4 | 2016 ControlEverything.com | GP7 | GND | GP6 | GP5 | A0 | A1 | GND | A2 | GP4 | SC | SCL | SDA | +5V | GND | MCP23008 | REV.E | ANSIO4R4xDPDT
